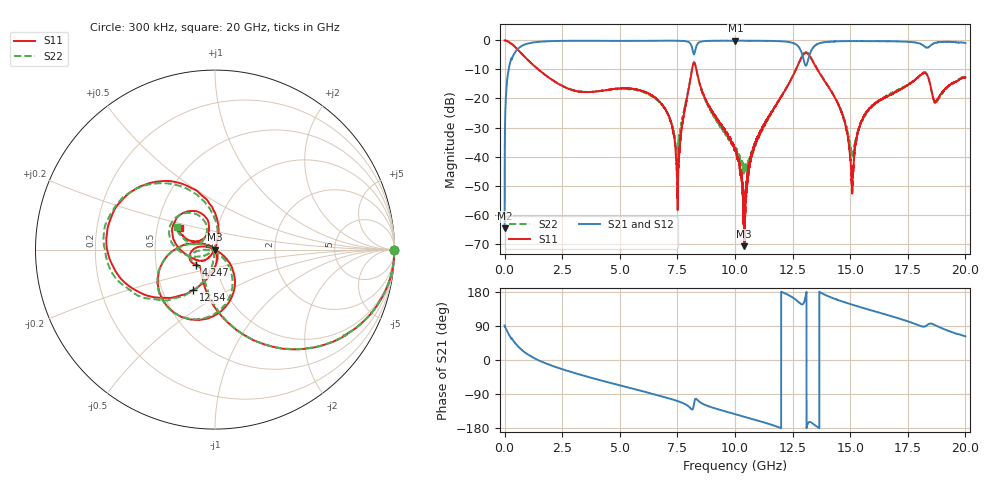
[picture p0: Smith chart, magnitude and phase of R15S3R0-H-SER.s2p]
!{R15S3R0}
!Johanson Technology Inc.
!www.johansontechnology.com
!Test Board Conditions:
!Substrate Type  RO4350B
!Substrate Thickness  20 mil
!Substrate Dk  3.66
!TL Type: GCPW
!TL Trace Width  34 mil
!TL Gap  10 mil
!Electrode orientation  Horizontal
!DUT TOPOLOGY	SERIES
!Mounting Pad LxW  26x52 mil
! Created Sat Feb  6 13:53:00 2021
# hz S ma R 50
! 2 Port Network Data from SP1.SP block
! freq  magS11  angS11  magS21  angS21  magS12  angS12  magS22  angS22
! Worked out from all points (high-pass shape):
!   20001 points, 300 kHz to 20 GHz, reference 50 ohm
!   highest |S21| = -0.08 dB at 10.02 GHz (marker M1); lowest = -64.8 dB at 300 kHz (marker M2)
!   |S21| within 3 dB of the highest: 551 MHz to 8.156 GHz (7.605 GHz wide, 175 % of centre); 13.34 GHz to end of sweep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
!   lowest |S11| = -70.9 dB at 10.4 GHz (marker M3), VSWR 1.00, Z = 50 - j0.0256 ohm
!   |S11| at or under -10 dB: 1.465 GHz to 8.133 GHz (6.669 GHz wide, 139 % of centre); 8.322 GHz to 12.65 GHz (4.326 GHz wide, 41.3 % of centre); 13.57 GHz to end of sweep
!   |S22| runs from -45.9 to 0.0 dB; largest |S21 - S12| = 0.013
!   S11 on the Smith chart (normalised r, x): 300 kHz: open; 4.247 GHz: 0.80, -0.14; 12.54 GHz: 0.71, -0.34; 20 GHz: 0.66, +0.17
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300000  1 -0.3  0.0005758 91.0  0.0005803 94.0  0.9984 -0.2
1.263e8  0.9712 -15.3  0.2343 74.4  0.2352 74.4  0.97 -15.3
4.383e8  0.7869 -43.6  0.6135 46.2  0.6147 46.3  0.7857 -43.4
1.3633e9  0.342 -87.8  0.9359 2.5  0.9357 2.4  0.342 -86.9
3.3343e9  0.1301 -129.1  0.9868 -39.5  0.9863 -39.6  0.1313 -129.3
4.2473e9  0.1364 -141.3  0.9856 -54.9  0.9845 -54.9  0.1359 -148.0
6.6673e9  0.09255 170.5  0.9876 -93.4  0.9883 -93.3  0.09136 -175.8
7.1983e9  0.04156 160.8  0.989 -102.5  0.9885 -102.5  0.0416 -178.4
7.5133e9  0.002472 -82.6  0.9868 -108.6  0.9881 -108.6  0.01361 -84.8
8.2413e9  0.4139 -130.0  0.5988 -108.7  0.5988 -108.4  0.4129 -132.0
1.00003e10  0.01249 133.2  0.989 -142.8  0.99 -142.8  0.01322 147.1
1.00213e10  0.0134 136.0  0.9912 -143.1  0.9891 -143.2  0.01352 145.7
1.04043e10  0.0002853 -116.2  0.9878 -149.7  0.9891 -149.7  0.006007 -174.6
1.09033e10  0.01765 -60.5  0.9873 -158.3  0.9883 -158.3  0.01655 -101.2
1.25363e10  0.255 -118.4  0.8997 163.7  0.905 163.8  0.2566 -118.0
1.30313e10  0.605 178.4  0.3898 158.7  0.3935 158.6  0.6087 -178.1
1.33343e10  0.467 125.0  0.6981 -165.8  0.6956 -166.0  0.4815 129.7
1.46073e10  0.06035 75.3  0.9692 155.5  0.9726 155.5  0.06154 78.6
1.50743e10  0.003658 150.0  0.978 146.2  0.973 146.4  0.01193 138.5
1.55433e10  0.04445 -126.7  0.9716 137.7  0.9779 137.8  0.04324 -148.7
1.66673e10  0.1123 -148.3  0.9713 117.7  0.9624 117.6  0.1158 -160.0
2e10  0.2303 148.5  0.9061 62.4  0.8994 62.0  0.2478 149.4
